(* Logix 5000 AddOnInstructionDefinition export ACS_FAULTS_ACTIVE; software revision 20.01 *)

TYPE DriveFaults :
STRUCT
   Positive_Limit : BOOL;   // Positive Limit
   Negative_Limit : BOOL;   // Negative Limit
   E_Stop : BOOL;   // E Stop
   Position_Error : BOOL;   // Position Error
   Feedback_Error : BOOL;   // Feedback Error
   Over_Current : BOOL;   // Overcurrent
   Motor_Over_Temperature : BOOL;   // Motor Over Temperature
   Drive_Over_Temperature : BOOL;   // Drive Over Temperature
   Drive_Over_Voltage : BOOL;   // Drive Over Voltage
   Drive_Under_Voltage : BOOL;   // Drive Under Voltage
   Flash_Error : BOOL;   // Flash Error
   I2T_Limit : BOOL;   // I2T Limit Fault
   Short_Circuit : BOOL;   // Short Circuit Fault
   Watchdog_Reset : BOOL;   // Watchdog Reset
END_STRUCT
END_TYPE

ADD_ON_INSTRUCTION ACS_FAULTS_ACTIVE   (* revision 2.0, vendor Tolomatic, Inc *)
// True if ACS Drive contains any faults
VAR_IN_OUT
   DriveFaults : DINT; {required}   // ACS.I.FAULTS
END_VAR
VAR
   LocalFaults : DriveFaults; {access None}   // Local Mapping for faults
END_VAR

ROUTINE Logic   (* ladder *)
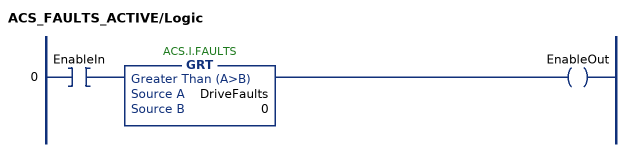
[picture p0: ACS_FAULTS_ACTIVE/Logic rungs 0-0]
   0: XIC(EnableIn)GRT(DriveFaults,0)OTE(EnableOut);
END_ROUTINE
END_ADD_ON_INSTRUCTION
